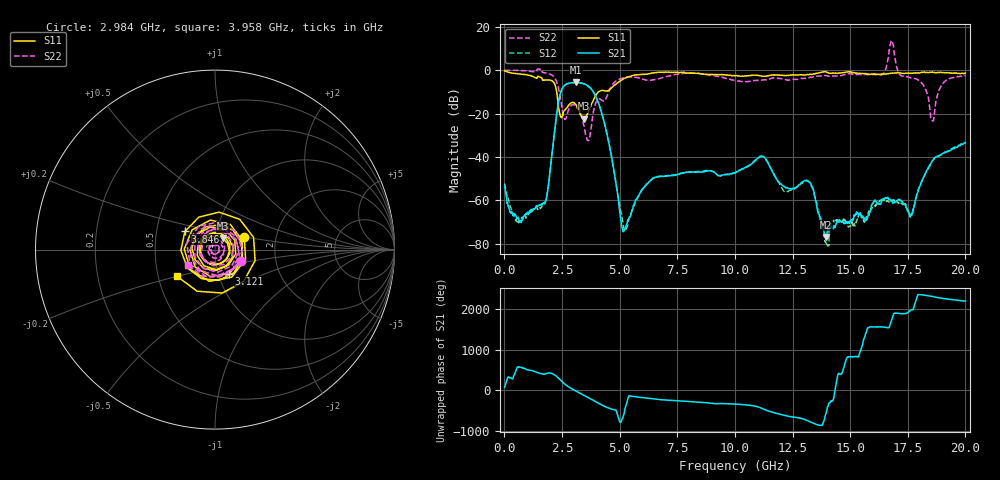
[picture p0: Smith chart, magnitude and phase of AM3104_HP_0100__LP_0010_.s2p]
!Created with skrf (http://scikit-rf.org).
# Hz S RI R 50.0
!freq ReS11 ImS11 ReS21 ImS21 ReS12 ImS12 ReS22 ImS22
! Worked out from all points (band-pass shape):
!   1601 points, 10 MHz to 20 GHz, reference 50 ohm
!   highest |S21| = -5.68 dB at 3.108 GHz (marker M1); lowest = -76.9 dB at 13.97 GHz (marker M2)
!   |S21| within 3 dB of the highest: 2.5 GHz to 3.771 GHz (1.271 GHz wide, 40.5 % of centre)
!   lowest |S11| = -22.3 dB at 3.458 GHz (marker M3), VSWR 1.17, Z = 54.1 + j6.9 ohm
!   |S11| at or under -10 dB: 2.269 GHz to 4.081 GHz (1.811 GHz wide, 57.1 % of centre)
!   |S22| runs from -32.5 to 13.7 dB; largest |S21 - S12| = 0.029
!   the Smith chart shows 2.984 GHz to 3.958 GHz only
!   S11 on the Smith chart (normalised r, x): 2.984 GHz: 1.37, +0.20; 3.121 GHz: 1.13, -0.31; 3.846 GHz: 0.70, +0.15; 3.958 GHz: 0.63, -0.20
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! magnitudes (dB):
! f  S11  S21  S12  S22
! 10 MHz  -0.3  -53.3  -52.3  0.0
! 572.2 MHz  -1.6  -68.2  -69.4  -0.1
! 1.684 GHz  -4.7  -61.3  -62.0  -1.1
! 2.409 GHz  -20.5  -11.6  -11.6  -11.4
! 2.984 GHz  -15.0  -5.7  -5.7  -16.0
! 3.108 GHz  -16.0  -5.7  -5.7  -16.7
! 3.121 GHz  -16.2  -5.7  -5.7  -16.9
! 3.346 GHz  -21.4  -6.0  -6.1  -20.8
! 3.458 GHz  -22.3  -6.3  -6.3  -25.8
! 3.846 GHz  -14.2  -9.8  -9.8  -20.2
! 3.958 GHz  -11.7  -12.0  -12.0  -15.3
! 5.17 GHz  -4.0  -74.3  -72.0  -3.5
! 6.682 GHz  -1.0  -49.1  -49.0  -4.0
! 10.01 GHz  -2.6  -47.4  -47.5  -4.8
! 11.18 GHz  -2.8  -39.7  -39.9  -4.6
! 13.34 GHz  -2.0  -53.5  -54.0  -3.3
! 13.97 GHz  -0.9  -76.9  -80.0  -2.6
! 16.68 GHz  -1.5  -59.6  -60.7  7.2
! 17.65 GHz  -1.4  -66.6  -66.6  -3.7
! 18.56 GHz  -0.9  -41.9  -41.9  -23.3
! 19.01 GHz  -1.1  -38.4  -38.6  -6.3
! 20 GHz  -1.4  -33.5  -33.2  -2.5
